| TEXAS INSTRUMENTS INCORPORATED
| Standard Linear and Logic Group
| IBIS Model of SN74CBT16390
| 16-BIT TO 32-BIT FET MULTIPLEXER/DEMULTIPLEXER BUS SWITCH
| This file contains package information for the following:
|  TSSOP 56-pin (DGG) package as [Component] CBT16390_DGG
|  TVSOP 56-pin (DGV) package as [Component] CBT16390_DGV
|  SSOP 56-pin (DL) package as [Component] CBT16390_DL
| This device can be powered at the following Vccs:
|  5 volt Vcc
| This file provides unique models under the [Model Selector] for each Vcc.
| For operation at a specific Vcc, select the appropriate model after each
| [Model Selector] keyword.
[IBIS Ver]   3.2
[Comment char]  |_char
[File Name]   sn74cbt16390.ibs
[File Rev]   1.0 | b_die
[Date]   June 25, 2002
[Source]   Data created from TI-SPICE simulations at TI-SLL.
[Notes]   The following is an IBIS list for the CBT16390.
   Please contact sllibis@ti.com with questions and
   comments concerning SLL IBIS models.
[Disclaimer] Property of Texas Instruments Incorporated.  Unauthorized
   reproduction and/or distribution is strictly prohibited.
   This product is protected under copyright law.
   Created  2002, (C) Copyright  2002, Texas Instruments
   Incorporated, All Rights Reserved
   UNLESS THERE IS A SIGNED, WRITTEN AGREEMENT TO THE
   CONTRARY, TEXAS INSTRUMENTS (TI) IS PROVIDING THE IBIS
   MODELS  AND WITHOUT ANY WARRANTY, EXPRESSED OR
   IMPLIED.  TI assumes no liability for:
   1) the accuracy of the IBIS models provided to your
   company;
   2) the proper functioning of these IBIS Models in your
   design or for any resulting applications; or
   3) infringement of patents, copyrights or intellectual
   property rights resulting from your use of these IBIS
   models.
   TI provides IBIS Models as a service to our customers.
   You and your company shall not distribute, sell or give
   these models to anyone else without prior written
   permission from TI.
   TI reserves the right to make changes to our products or
   to discontinue any semiconductor product or service
   without notice, and advises our customers to obtain the
   latest version of relevant information to verify, before
   placing orders, that the information being relied on is
   current.
   Please be aware that your receipt and use of the IBIS
   information provided shall serve as acceptance of these
   terms and conditions.  If you do not accept these terms,
   you should return or destroy the IBIS models and any
   other accompanying information immediately.
| Component CBT16390_DGG 56-pin TSSOP
[Component]   CBT16390_DGG
[Manufacturer]   Texas Instruments, Inc.
[Package]
|   typ   min   max
R_pkg   4.500e-02   3.500e-02   6.200e-02
L_pkg   3.324e-09   2.403e-09   5.094e-09
C_pkg   5.640e-13   3.410e-13   9.140e-13
[Pin]   signal_name   model_name   R_pin   L_pin   C_pin
1   A1   CBT16390_IO   6.200e-02   5.094e-09   8.560e-13
2   2B1   CBT16390_IO   6.100e-02   4.621e-09   9.020e-13
3   2B2   CBT16390_IO   6.000e-02   4.316e-09   8.020e-13
4   A3   CBT16390_IO   5.900e-02   3.968e-09   6.980e-13
5   2B3   CBT16390_IO   5.700e-02   3.716e-09   6.490e-13
6   2B4   CBT16390_IO   4.200e-02   3.517e-09   6.520e-13
7   A5   CBT16390_IO   4.100e-02   3.160e-09   5.700e-13
8   2B5   CBT16390_IO   3.900e-02   2.981e-09   4.820e-13
9   2B6   CBT16390_IO   3.900e-02   2.809e-09   4.470e-13
10   A7   CBT16390_IO   3.800e-02   2.715e-09   4.090e-13
11   2B7   CBT16390_IO   4.100e-02   2.675e-09   3.910e-13
12   2B8   CBT16390_IO   3.900e-02   2.536e-09   3.660e-13
13   GND   GND   3.900e-02   2.457e-09   3.480e-13
14   VCC   POWER   3.800e-02   2.411e-09   3.530e-13
15   A9   CBT16390_IO   3.900e-02   2.456e-09   3.550e-13
16   2B9   CBT16390_IO   3.900e-02   2.471e-09   3.490e-13
17   2B10   CBT16390_IO   4.000e-02   2.580e-09   3.700e-13
18   A11   CBT16390_IO   3.800e-02   2.651e-09   3.890e-13
19   2B11   CBT16390_IO   3.800e-02   2.739e-09   4.110e-13
20   2B12   CBT16390_IO   3.900e-02   2.838e-09   4.490e-13
21   A13   CBT16390_IO   3.800e-02   2.988e-09   4.840e-13
22   2B13   CBT16390_IO   3.800e-02   3.105e-09   5.640e-13
23   2B14   CBT16390_IO   4.000e-02   3.427e-09   6.380e-13
24   A15   CBT16390_IO   5.600e-02   3.654e-09   6.410e-13
25   2B15   CBT16390_IO   5.700e-02   3.932e-09   7.000e-13
26   2B16   CBT16390_IO   5.800e-02   4.257e-09   8.060e-13
27   NC   NC   5.700e-02   4.580e-09   9.140e-13
28   NC   NC   5.900e-02   5.038e-09   8.610e-13
29   NOE2   CBT16390_NOE   6.000e-02   5.058e-09   8.580e-13
30   NOE1   CBT16390_NOE   5.600e-02   4.543e-09   9.040e-13
31   A16   CBT16390_IO   5.700e-02   4.240e-09   8.030e-13
32   1B16   CBT16390_IO   5.700e-02   3.929e-09   7.000e-13
33   1B15   CBT16390_IO   5.600e-02   3.616e-09   6.370e-13
34   A14   CBT16390_IO   3.700e-02   3.368e-09   6.400e-13
35   1B14   CBT16390_IO   3.600e-02   3.024e-09   5.630e-13
36   1B13   CBT16390_IO   3.500e-02   2.876e-09   4.740e-13
37   A12   CBT16390_IO   3.500e-02   2.745e-09   4.440e-13
38   1B12   CBT16390_IO   3.700e-02   2.683e-09   4.050e-13
39   1B11   CBT16390_IO   3.800e-02   2.603e-09   3.820e-13
40   A10   CBT16390_IO   3.800e-02   2.510e-09   3.620e-13
41   1B10   CBT16390_IO   3.600e-02   2.412e-09   3.410e-13
42   1B9   CBT16390_IO   3.800e-02   2.416e-09   3.490e-13
43   VCC   POWER   3.700e-02   2.403e-09   3.490e-13
44   GND   GND   3.700e-02   2.429e-09   3.410e-13
45   A8   CBT16390_IO   3.600e-02   2.482e-09   3.580e-13
46   1B8   CBT16390_IO   3.700e-02   2.615e-09   3.810e-13
47   1B7   CBT16390_IO   3.500e-02   2.669e-09   4.020e-13
48   A6   CBT16390_IO   3.600e-02   2.763e-09   4.420e-13
49   1B6   CBT16390_IO   3.600e-02   2.942e-09   4.780e-13
50   1B5   CBT16390_IO   3.500e-02   3.053e-09   5.640e-13
51   A4   CBT16390_IO   3.600e-02   3.409e-09   6.410e-13
52   1B4   CBT16390_IO   5.800e-02   3.698e-09   6.410e-13
53   1B3   CBT16390_IO   5.900e-02   3.975e-09   6.970e-13
54   A2   CBT16390_IO   6.100e-02   4.327e-09   8.020e-13
55   1B2   CBT16390_IO   6.100e-02   4.624e-09   9.050e-13
56   1B1   CBT16390_IO   6.000e-02   5.063e-09   8.580e-13
| Component CBT16390_DGV 56-pin TVSOP
[Component]   CBT16390_DGV
[Manufacturer]   Texas Instruments, Inc.
[Package]
|   typ   min   max
R_pkg   6.300e-02   5.000e-02   8.600e-02
L_pkg   2.945e-09   2.392e-09   3.938e-09
C_pkg   3.910e-13   2.710e-13   5.880e-13
[Pin]   signal_name   model_name   R_pin   L_pin   C_pin
1   A1   CBT16390_IO   6.800e-02   3.933e-09   5.880e-13
2   2B1   CBT16390_IO   6.800e-02   3.569e-09   5.860e-13
3   2B2   CBT16390_IO   7.600e-02   3.464e-09   5.150e-13
4   A3   CBT16390_IO   8.600e-02   3.451e-09   4.580e-13
5   2B3   CBT16390_IO   8.200e-02   3.278e-09   4.260e-13
6   2B4   CBT16390_IO   7.700e-02   3.143e-09   3.870e-13
7   A5   CBT16390_IO   6.900e-02   2.971e-09   4.010e-13
8   2B5   CBT16390_IO   5.000e-02   2.787e-09   3.790e-13
9   2B6   CBT16390_IO   5.100e-02   2.686e-09   3.200e-13
10   A7   CBT16390_IO   5.200e-02   2.607e-09   3.160e-13
11   2B7   CBT16390_IO   5.300e-02   2.497e-09   2.970e-13
12   2B8   CBT16390_IO   5.400e-02   2.438e-09   2.920e-13
13   GND   GND   5.500e-02   2.412e-09   2.860e-13
14   VCC   POWER   5.500e-02   2.400e-09   2.730e-13
15   A9   CBT16390_IO   5.500e-02   2.402e-09   2.730e-13
16   2B9   CBT16390_IO   5.400e-02   2.398e-09   2.840e-13
17   2B10   CBT16390_IO   5.400e-02   2.407e-09   2.890e-13
18   A11   CBT16390_IO   5.300e-02   2.448e-09   2.930e-13
19   2B11   CBT16390_IO   5.200e-02   2.548e-09   3.110e-13
20   2B12   CBT16390_IO   5.100e-02   2.623e-09   3.160e-13
21   A13   CBT16390_IO   5.000e-02   2.725e-09   3.700e-13
22   2B13   CBT16390_IO   6.500e-02   2.903e-09   3.940e-13
23   2B14   CBT16390_IO   7.300e-02   3.086e-09   3.870e-13
24   A15   CBT16390_IO   8.200e-02   3.272e-09   4.280e-13
25   2B15   CBT16390_IO   8.200e-02   3.394e-09   4.570e-13
26   2B16   CBT16390_IO   7.100e-02   3.374e-09   5.080e-13
27   NC   NC   6.900e-02   3.572e-09   5.810e-13
28   NC   NC   6.900e-02   3.937e-09   5.740e-13
29   NOE2   CBT16390_NOE   6.900e-02   3.923e-09   5.690e-13
30   NOE1   CBT16390_NOE   6.800e-02   3.546e-09   5.740e-13
31   A16   CBT16390_IO   7.400e-02   3.422e-09   5.180e-13
32   1B16   CBT16390_IO   8.100e-02   3.395e-09   4.680e-13
33   1B15   CBT16390_IO   8.000e-02   3.255e-09   4.310e-13
34   A14   CBT16390_IO   7.100e-02   3.063e-09   3.860e-13
35   1B14   CBT16390_IO   6.100e-02   2.878e-09   3.900e-13
36   1B13   CBT16390_IO   5.000e-02   2.709e-09   3.640e-13
37   A12   CBT16390_IO   5.100e-02   2.607e-09   3.110e-13
38   1B12   CBT16390_IO   5.100e-02   2.532e-09   3.060e-13
39   1B11   CBT16390_IO   5.300e-02   2.440e-09   2.890e-13
40   A10   CBT16390_IO   5.300e-02   2.399e-09   2.860e-13
41   1B10   CBT16390_IO   5.400e-02   2.392e-09   2.820e-13
42   1B9   CBT16390_IO   5.500e-02   2.399e-09   2.710e-13
43   VCC   POWER   5.500e-02   2.395e-09   2.710e-13
44   GND   GND   5.500e-02   2.403e-09   2.830e-13
45   A8   CBT16390_IO   5.400e-02   2.421e-09   2.880e-13
46   1B8   CBT16390_IO   5.300e-02   2.472e-09   2.920e-13
47   1B7   CBT16390_IO   5.100e-02   2.569e-09   3.090e-13
48   A6   CBT16390_IO   5.100e-02   2.636e-09   3.130e-13
49   1B6   CBT16390_IO   5.000e-02   2.739e-09   3.660e-13
50   1B5   CBT16390_IO   6.500e-02   2.922e-09   3.900e-13
51   A4   CBT16390_IO   7.200e-02   3.076e-09   3.840e-13
52   1B4   CBT16390_IO   8.100e-02   3.249e-09   4.300e-13
53   1B3   CBT16390_IO   8.300e-02   3.400e-09   4.550e-13
54   A2   CBT16390_IO   7.300e-02   3.421e-09   5.060e-13
55   1B2   CBT16390_IO   6.900e-02   3.579e-09   5.780e-13
56   1B1   CBT16390_IO   6.900e-02   3.938e-09   5.810e-13
| Component CBT16390_DL 56-pin SSOP
[Component]   CBT16390_DL
[Manufacturer]   Texas Instruments, Inc.
[Package]
|   typ   min   max
R_pkg   5.500e-02   4.800e-02   6.700e-02
L_pkg   6.539e-09   4.802e-09   9.746e-09
C_pkg   1.880e-13   7.600e-14   5.170e-13
[Pin]   signal_name   model_name   R_pin   L_pin   C_pin
1   A1   CBT16390_IO   6.400e-02   9.646e-09   5.130e-13
2   2B1   CBT16390_IO   5.900e-02   8.723e-09   2.700e-13
3   2B2   CBT16390_IO   5.900e-02   8.139e-09   2.230e-13
4   A3   CBT16390_IO   5.600e-02   7.554e-09   2.010e-13
5   2B3   CBT16390_IO   5.400e-02   6.991e-09   1.950e-13
6   2B4   CBT16390_IO   5.300e-02   6.659e-09   2.020e-13
7   A5   CBT16390_IO   5.500e-02   6.321e-09   2.070e-13
8   2B5   CBT16390_IO   5.500e-02   5.942e-09   1.330e-13
9   2B6   CBT16390_IO   5.700e-02   5.767e-09   1.320e-13
10   A7   CBT16390_IO   5.400e-02   5.459e-09   1.210e-13
11   2B7   CBT16390_IO   5.100e-02   5.224e-09   1.400e-13
12   2B8   CBT16390_IO   4.800e-02   5.088e-09   1.260e-13
13   GND   GND   5.000e-02   5.021e-09   9.600e-14
14   VCC   POWER   5.100e-02   4.802e-09   7.600e-14
15   A9   CBT16390_IO   5.100e-02   4.803e-09   7.600e-14
16   2B9   CBT16390_IO   5.000e-02   5.021e-09   9.600e-14
17   2B10   CBT16390_IO   4.800e-02   5.088e-09   1.260e-13
18   A11   CBT16390_IO   5.100e-02   5.224e-09   1.400e-13
19   2B11   CBT16390_IO   5.400e-02   5.459e-09   1.210e-13
20   2B12   CBT16390_IO   5.700e-02   5.768e-09   1.330e-13
21   A13   CBT16390_IO   5.500e-02   5.942e-09   1.330e-13
22   2B13   CBT16390_IO   5.500e-02   6.320e-09   2.060e-13
23   2B14   CBT16390_IO   5.300e-02   6.659e-09   2.030e-13
24   A15   CBT16390_IO   5.400e-02   6.991e-09   1.960e-13
25   2B15   CBT16390_IO   5.600e-02   7.554e-09   2.010e-13
26   2B16   CBT16390_IO   5.900e-02   8.139e-09   2.230e-13
27   NC   NC   5.900e-02   8.727e-09   2.700e-13
28   NC   NC   6.700e-02   9.746e-09   5.170e-13
29   NOE2   CBT16390_NOE   6.300e-02   9.630e-09   5.110e-13
30   NOE1   CBT16390_NOE   6.000e-02   8.751e-09   2.710e-13
31   A16   CBT16390_IO   6.000e-02   8.184e-09   2.250e-13
32   1B16   CBT16390_IO   5.600e-02   7.543e-09   2.000e-13
33   1B15   CBT16390_IO   5.400e-02   7.005e-09   1.960e-13
34   A14   CBT16390_IO   5.600e-02   6.714e-09   2.040e-13
35   1B14   CBT16390_IO   5.800e-02   6.384e-09   2.080e-13
36   1B13   CBT16390_IO   5.700e-02   5.976e-09   1.340e-13
37   A12   CBT16390_IO   5.700e-02   5.743e-09   1.300e-13
38   1B12   CBT16390_IO   5.400e-02   5.468e-09   1.190e-13
39   1B11   CBT16390_IO   5.500e-02   5.328e-09   1.420e-13
40   A10   CBT16390_IO   5.200e-02   5.189e-09   1.290e-13
41   1B10   CBT16390_IO   5.200e-02   5.053e-09   9.600e-14
42   1B9   CBT16390_IO   5.100e-02   4.825e-09   7.600e-14
43   VCC   POWER   5.400e-02   4.896e-09   7.800e-14
44   GND   GND   5.200e-02   5.093e-09   9.700e-14
45   A8   CBT16390_IO   5.100e-02   5.179e-09   1.280e-13
46   1B8   CBT16390_IO   5.400e-02   5.314e-09   1.420e-13
47   1B7   CBT16390_IO   5.500e-02   5.511e-09   1.210e-13
48   A6   CBT16390_IO   5.700e-02   5.771e-09   1.310e-13
49   1B6   CBT16390_IO   5.600e-02   5.957e-09   1.330e-13
50   1B5   CBT16390_IO   5.500e-02   6.320e-09   2.060e-13
51   A4   CBT16390_IO   5.200e-02   6.621e-09   2.000e-13
52   1B4   CBT16390_IO   5.300e-02   6.973e-09   1.950e-13
53   1B3   CBT16390_IO   5.700e-02   7.571e-09   2.020e-13
54   A2   CBT16390_IO   5.700e-02   8.097e-09   2.220e-13
55   1B2   CBT16390_IO   5.900e-02   8.723e-09   2.710e-13
56   1B1   CBT16390_IO   6.100e-02   9.560e-09   5.090e-13
[Series Switch Groups]
| Function Group States
On  1 /   | A1-A16->1B1-1B16 NOE1 LOW, NOE2 HIGH
On  2 /   | A1-A16->2B1-2B16 NOE1 HIGH, NOE2 LOW
On  1 2 /   | Enable Both
[Series Pin Mapping]   pin_2   model_name   function_table_group
1   56   CBT16390_IO_S   1
4   53   CBT16390_IO_S   1
7   50   CBT16390_IO_S   1
10   47   CBT16390_IO_S   1
15   42   CBT16390_IO_S   1
18   39   CBT16390_IO_S   1
21   36   CBT16390_IO_S   1
24   33   CBT16390_IO_S   1
31   32   CBT16390_IO_S   1
34   35   CBT16390_IO_S   1
37   38   CBT16390_IO_S   1
40   41   CBT16390_IO_S   1
45   46   CBT16390_IO_S   1
48   49   CBT16390_IO_S   1
51   52   CBT16390_IO_S   1
54   55   CBT16390_IO_S   1
1   2   CBT16390_IO_S   2
4   5   CBT16390_IO_S   2
7   8   CBT16390_IO_S   2
10   11   CBT16390_IO_S   2
15   16   CBT16390_IO_S   2
18   19   CBT16390_IO_S   2
21   22   CBT16390_IO_S   2
24   25   CBT16390_IO_S   2
31   26   CBT16390_IO_S   2
34   23   CBT16390_IO_S   2
37   20   CBT16390_IO_S   2
40   17   CBT16390_IO_S   2
45   12   CBT16390_IO_S   2
48   9   CBT16390_IO_S   2
51   6   CBT16390_IO_S   2
54   3   CBT16390_IO_S   2
[Model]   CBT16390_IO_S
Model_type  Series_switch
| variable   typ   min   max
C_comp   0   0   0
[Temperature Range]   40   100   -40
| Ambient temperature   25   85   -40
[Voltage range]   5   4.5   5.5
[On]
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[Off]
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| Models and submodels in the file (3): CBT16390_NOE (Input), CBT16390_IO_S (Series_switch), CBT16390_IO (Terminator)
